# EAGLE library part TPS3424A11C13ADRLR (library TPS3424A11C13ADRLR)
Supervisory Circuits Nanopower push-button controller with programmable delay Source: Datasheet
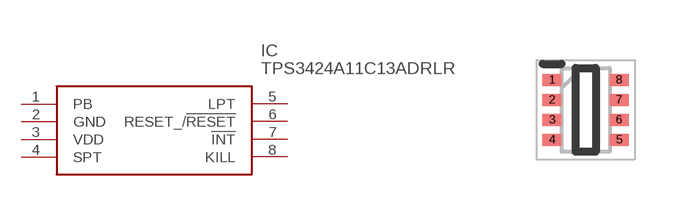
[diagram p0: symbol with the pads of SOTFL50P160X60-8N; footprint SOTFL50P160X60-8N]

Designator prefix IC

## TPS3424A11C13ADRLR (Description: Supervisory Circuits Nanopower push-button controller with programmable delay; Height: 0.6mm; Manufacturer_Name: Texas Instruments; Manufacturer_Part_Number: TPS3424A11C13ADRLR)  [SOTFL50P160X60-8N]
1  PB
2  GND
3  VDD
4  SPT
5  LPT
6  RESET_/!RESET
7  !INT
8  KILL

## Footprint SOTFL50P160X60-8N (pad centres in mm)
DRL0008A
smd 0.475 x 0.3: 1 -0.838,0.75; 2 -0.838,0.25; 3 -0.838,-0.25; 4 -0.838,-0.75; 5 0.838,-0.75; 6 0.838,-0.25; 7 0.838,0.25; 8 0.838,0.75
